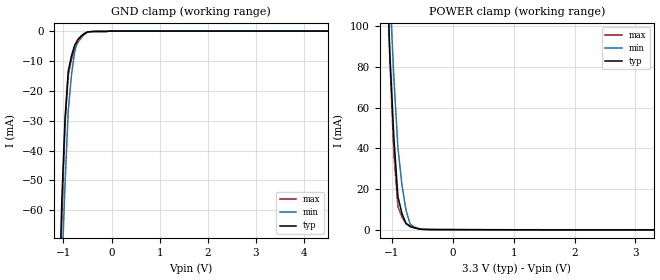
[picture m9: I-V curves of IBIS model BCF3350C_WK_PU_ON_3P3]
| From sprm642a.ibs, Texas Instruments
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|BCF3350C_WK_PD_ON_3P3; WEAK_PULLDOWN_ON
|   Model Cell BCF3350C_WK_PU_ON_3P3
|BCF3350C_WK_PU_ON_3P3
[Model]   BCF3350C_WK_PU_ON_3P3
Model_type   Input
Polarity   Non-Inverting
Vinl =  0.8
Vinh =  2
C_comp   1.081618p   0.946736p   1.221412p
[Model Spec]
Vinl   0.8   0.8   0.8
Vinh   2   2   2
[Temperature Range]   25   155   -40
[Voltage Range]   3.3   2.97   3.63
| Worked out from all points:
|   GND clamp passes 1 mA (typ) near -0.58 V on its own axis
|   POWER clamp passes 1 mA (typ) near -0.65 V on its own axis
| Nom Voltages:
|   VDD=1.2, VDDS=3.3, VSS=0
| Min Voltages:
|   VDD=1.08, VDDS=2.97, VSS=0
| Max Voltages:
|   VDD=1.32, VDDS=3.63, VSS=0
[POWER_clamp]
|   voltage   I(typ)   I(min)   I(max)
-3.3V     2.318A     2.595A     3.049A
-1.1V     141.5mA    168mA      152.4mA
-1.033V   87.22mA    117.8mA    84.46mA
-966.7mV  45.45mA    75.19mA    37.43mA
-900mV    16.24mA    40.27mA    11.28mA
-833.3mV  7.9mA      21.98mA    6.136mA
-766.7mV  2.98mA     9.488mA    3.023mA
-700mV    1.481mA    2.786mA    1.936mA
-566.7mV  418.3uA    505.1uA    545.1uA
-366.7mV  37.54uA    32.82uA    50.64uA
3.3V      -108.8uA   -58.67uA   -174uA
[GND_clamp]
|   voltage   I(typ)   I(min)   I(max)
-3.3V     -1.888A    -1.585A    -3.154A
-1.1V     -95.8mA    -113.9mA   -112.1mA
-1.033V   -56.72mA   -80.31mA   -63.63mA
-966.7mV  -29.27mA   -51.24mA   -31.19mA
-900mV    -13.44mA   -26.69mA   -14.78mA
-833.3mV  -8.296mA   -14.8mA    -9.57mA
-766.7mV  -4.761mA   -6.885mA   -5.913mA
-700mV    -2.841mA   -2.943mA   -3.814mA
-566.7mV  -850.9uA   -829.9uA   -1.14mA
-500mV    -297.8uA   -331.1uA   -390.3uA
-33.33mV  0A         0A         0A
6.6V      0A         0A         0A
